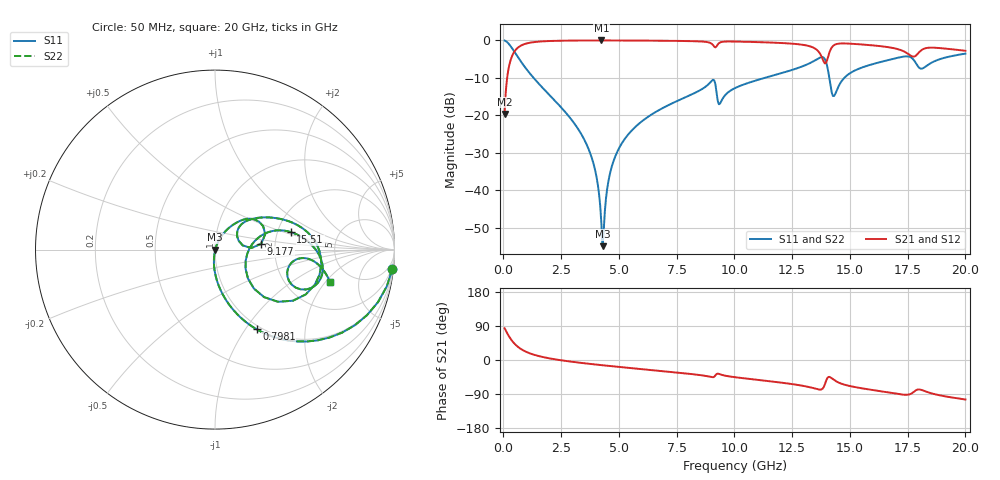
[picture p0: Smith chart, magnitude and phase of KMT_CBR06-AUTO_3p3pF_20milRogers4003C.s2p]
! Data measured by Modelithics Inc. support@modelithics.com 813-866-6335
! KEMET CBR06-AUTO 3.3pF, Pad Width= 0.851mm, Pad Length= 0.64mm, Pad Gap= 0.62mm, 20mil Rogers 4003C substrate Data, January 2022
# hz S ma R 50
! 2 Port Network Data from SP1.SP block
! freq  magS11  angS11  magS21  angS21  magS12  angS12  magS22  angS22
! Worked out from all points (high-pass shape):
!   401 points, 50 MHz to 20 GHz, reference 50 ohm
!   highest |S21| = -0.02 dB at 4.239 GHz (marker M1); lowest = -19.6 dB at 50 MHz (marker M2)
!   |S21| within 3 dB of the highest: 473.4 MHz to 13.64 GHz (13.17 GHz wide, 187 % of centre); 14.13 GHz to 17.36 GHz (3.237 GHz wide, 20.6 % of centre)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
!   lowest |S11| = -54.9 dB at 4.289 GHz (marker M3), VSWR 1.00, Z = 50.2 - j0.0871 ohm
!   |S11| at or under -10 dB: 1.306 GHz to 11.31 GHz (10.01 GHz wide, 159 % of centre); 14.11 GHz to 14.76 GHz (649 MHz wide, 4.5 % of centre)
!   |S22| runs from -54.9 to 0.0 dB; largest |S21 - S12| = 0
!   S11 on the Smith chart (normalised r, x): 50 MHz: 1, -19; 798.1 MHz: 0.95, -1.13; 9.177 GHz: 1.69, +0.12; 15.51 GHz: 2.37, +0.57; 20 GHz: 3.44, -2.24
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5e7  0.9945 -6.1  0.1041 83.8  0.1041 83.8  0.9945 -6.1
2.99375e8  0.8458 -33.2  0.5326 56.8  0.5326 56.8  0.8458 -33.2
7.98125e8  0.5006 -62.4  0.8648 27.5  0.8648 27.5  0.5006 -62.4
3.391625e9  0.05476 -96.2  0.9968 -7.8  0.9968 -7.8  0.05476 -96.2
3.94025e9  0.02025 -96.9  0.998 -11.6  0.998 -11.6  0.02025 -96.9
4.2395e9  0.003636 -75.1  0.9981 -13.5  0.9981 -13.5  0.003636 -75.1
4.289375e9  0.001802 -28.8  0.9981 -13.8  0.9981 -13.8  0.001802 -28.8
4.588625e9  0.01555 67.6  0.9979 -15.7  0.9979 -15.7  0.01555 67.6
4.987625e9  0.03565 68.8  0.9973 -18.1  0.9973 -18.1  0.03565 68.8
6.73325e9  0.1176 60.4  0.9904 -28.4  0.9904 -28.4  0.1176 60.4
9.177125e9  0.2592 7.2  0.8064 -40.4  0.8064 -40.4  0.2592 7.2
9.376625e9  0.144 30.9  0.9381 -37.7  0.9381 -37.7  0.144 30.9
1.0025e10  0.2312 42.7  0.965 -45.4  0.965 -45.4  0.2312 42.7
1.336662e10  0.5157 11.8  0.814 -73.3  0.814 -73.3  0.5157 11.8
1.376562e10  0.5983 -8.6  0.6145 -77.6  0.6145 -77.6  0.5983 -8.6
1.396512e10  0.519 -33.3  0.4998 -55.6  0.4998 -55.6  0.519 -33.3
1.431425e10  0.1812 -7.3  0.8639 -52.7  0.8639 -52.7  0.1812 -7.3
1.551125e10  0.4336 13.0  0.8827 -74.6  0.8827 -74.6  0.4336 13.0
1.670825e10  0.5512 1.3  0.8079 -86.0  0.8079 -86.0  0.5512 1.3
1.745638e10  0.6125 -12.9  0.6805 -91.8  0.6805 -91.8  0.6125 -12.9
1.805488e10  0.4215 -17.4  0.7236 -78.2  0.7236 -78.2  0.4215 -17.4
2e10  0.666 -15.8  0.7272 -104.2  0.7272 -104.2  0.666 -15.8
